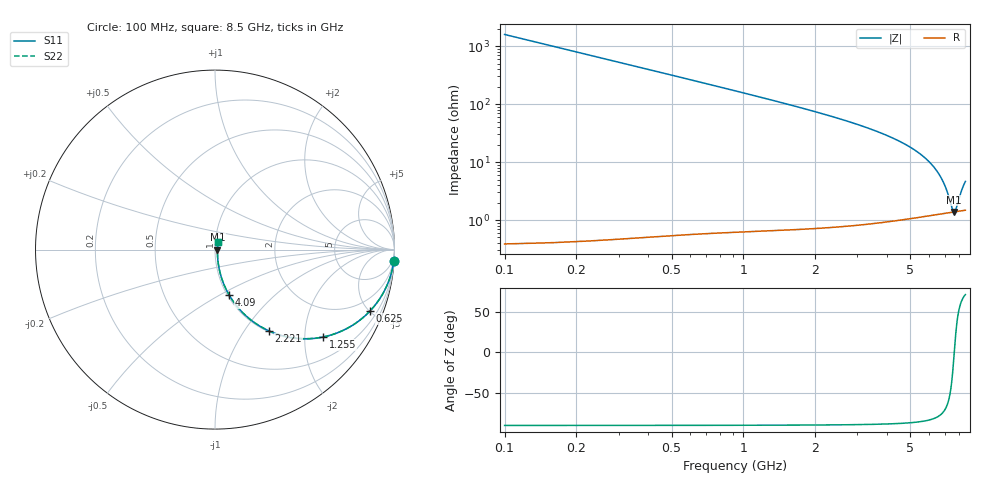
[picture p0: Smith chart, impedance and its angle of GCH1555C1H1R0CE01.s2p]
!Murata Part Number: GCH1555C1H1R0CE01
!These Parameters are Measured in Series Mode Connection
!Data Generated on Jun 19, 2026
!  o--ll--o
!Port1  Port2
!  o------o
!Operation Temp=25[degC], DC Bias Voltage=0[V]
!Freq. Start=100[MHz] Stop=9[GHz] 401[Steps]
# Hz S RI R 50
!Freq.(Hz) S11(Real) S11(Imag) S21(Real) S21(Imag) S12(Real) S12(Imag) S22(Real) S22(Imag)
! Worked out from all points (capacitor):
!   401 points, 100 MHz to 8.5 GHz, reference 50 ohm
!   read as one part in series: C = 1 pF near 142 MHz
!   lowest |Z| = 1.38 ohm at 7.618 GHz (marker M1)
!   series resonance near 7.633 GHz, so ESL is about 430 pH
!   S11 on the Smith chart (normalised r, x): 100 MHz: 1, -32; 625 MHz: 1.01, -5.06; 1.255 GHz: 1.01, -2.46; 2.221 GHz: 1.01, -1.31; 4.09 GHz: 1.02, -0.55; 8.5 GHz: 1.03, +0.09
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1e8  0.9961 -0.0626  0.00395 0.0626  0.00395 0.0626  0.9961 -0.0626
2.05e8  0.9836 -0.1268  0.0164 0.1268  0.0164 0.1268  0.9836 -0.1268
3.1e8  0.9632 -0.1879  0.0368 0.1879  0.0368 0.1879  0.9632 -0.1879
4.57e8  0.9229 -0.266  0.0771 0.266  0.0771 0.266  0.9229 -0.266
6.25e8  0.8641 -0.3416  0.1359 0.3416  0.1359 0.3416  0.8641 -0.3416
8.98e8  0.7523 -0.43  0.2477 0.43  0.2477 0.43  0.7523 -0.43
1.255e9  0.6024 -0.4868  0.3976 0.4868  0.3976 0.4868  0.6024 -0.4868
1.507e9  0.5065 -0.4967  0.4935 0.4967  0.4935 0.4967  0.5065 -0.4967
2.221e9  0.3016 -0.4534  0.6984 0.4534  0.6984 0.4534  0.3016 -0.4534
2.914e9  0.1817 -0.377  0.8183 0.377  0.8183 0.377  0.1817 -0.377
4.09e9  0.0779 -0.2515  0.9221 0.2515  0.9221 0.2515  0.0779 -0.2515
4.3e9  0.067 -0.2315  0.933 0.2315  0.933 0.2315  0.067 -0.2315
5.707e9  0.0254 -0.117  0.9746 0.117  0.9746 0.117  0.0254 -0.117
6.148e9  0.0196 -0.0869  0.9804 0.0869  0.9804 0.0869  0.0196 -0.0869
6.526e9  0.0163 -0.0628  0.9837 0.0628  0.9837 0.0628  0.0163 -0.0628
6.841e9  0.0147 -0.0438  0.9853 0.0438  0.9853 0.0438  0.0147 -0.0438
7.114e9  0.0138 -0.0281  0.9862 0.0281  0.9862 0.0281  0.0138 -0.0281
7.492e9  0.0135 -0.00745  0.9865 0.00745  0.9865 0.00745  0.0135 -0.00745
7.618e9  0.0136 -0.000804  0.9864 0.000804  0.9864 0.000804  0.0136 -0.000804
7.744e9  0.0138 0.00573  0.9862 -0.00573  0.9862 -0.00573  0.0138 0.00573
8.164e9  0.0149 0.0267  0.9851 -0.0267  0.9851 -0.0267  0.0149 0.0267
8.5e9  0.0164 0.0427  0.9836 -0.0427  0.9836 -0.0427  0.0164 0.0427
